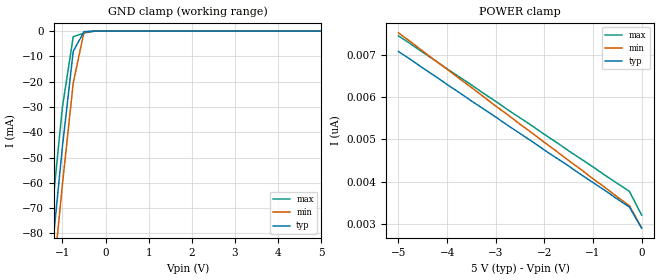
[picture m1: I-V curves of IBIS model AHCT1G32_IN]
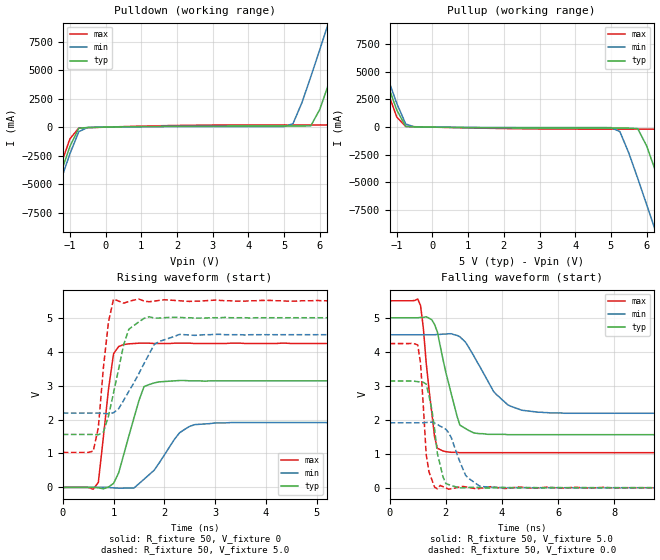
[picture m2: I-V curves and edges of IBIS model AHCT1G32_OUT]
| TEXAS INSTRUMENTS INCORPORATED
| Standard Linear and Logic Group
| IBIS Model of SN74AHCT1G32
| SINGLE 2-INPUT POSITIVE-NOR GATE
| SOT 5-pin (DCK) and SOT 5-pin (DBV) Package
[IBIS Ver]   3.2
[Comment Char]  |_char
[File Name]   ahct1g32.ibs
[File Rev]   2.0 J_die
[Date]   May 24, 2000
[Source]   Data created from HSPICE simulations at TI-SLL.
[Notes]   The following is an IBIS list for the AHCT1G32.
|   Please contact sllibis@ti.com with questions and
|   comments concerning SLL IBIS models.
[Disclaimer] Property of Texas Instruments Incorporated.  Unauthorized
   reproduction and/or distribution is strictly prohibited.
   This product is protected under copyright law.
   Created 2000, (C) Copyright 2000, Texas Instruments Inc.,
   All Rights Reserved.
   UNLESS THERE IS A SIGNED, WRITTEN AGREEMENT TO THE
   CONTRARY, TEXAS INSTRUMENTS () IS PROVIDING THE IBIS
   MODELS  AND WITHOUT ANY WARRANTY, EXPRESSED OR
   IMPLIED.  TI assumes no liability for:
   1) the accuracy of the IBIS models provided to your
   company;
   2) the proper functioning of these IBIS Models in your
   design or for any resulting applications; or
   3) infringement of patents, copyrights or intellectual
   property rights resulting from your use of these IBIS
   models.
   TI provides IBIS Models as a service to our customers.
   You and your company shall not distribute, sell or give
   these models to anyone else without prior written
   permission from TI.
   TI reserves the right to make changes to our products or
   to discontinue any semiconductor product or service
   without notice, and advises our customers to obtain the
   latest version of relevant information to verify, before
   placing orders, that the information being relied on is
   current.
   Please be aware that your receipt and use of the IBIS
   information provided shall serve as acceptance of these
   terms and conditions.  If you do not accept these terms,
   you should return or destroy the IBIS models and any
   other accompanying information immediately.
|   Component AHCT1G32_DCK
[Component]   AHCT1G32_DCK
[Manufacturer]  Texas Instruments, Inc.
[Package]
|   typ   min   max
R_pkg   0.020   0.017   0.025
L_pkg   0.998nH   0.881nH   1.069nH
C_pkg   0.146pF   0.118pF   0.205pF
[Pin]   signal_name   model_name   R_pin   L_pin   C_pin
1   A   AHCT1G32_IN   0.019   1.069nH   0.162pF
2   B   AHCT1G32_IN   0.018   0.881nH   0.121pF
3   GND   GND   0.017   1.031nH   0.205pF
4   Y   AHCT1G32_OUT   0.020   0.960nH   0.124pF
5   VCC   POWER   0.025   1.049nH   0.118pF
|   Component AHCT1G32_DBV
[Component]   AHCT1G32_DBV
[Manufacturer]  Texas Instruments, Inc.
[Package]
|   typ   min   max
R_pkg   0.025   0.021   0.029
L_pkg   1.529nH   1.312nH   1.906nH
C_pkg   0.156pF   0.110pF   0.240pF
[Pin]   signal_name   model_name   R_pin   L_pin   C_pin
1   A   AHCT1G32_IN   0.021   1.511nH   0.144pF
2   B   AHCT1G32_IN   0.023   1.312nH   0.138pF
3   GND   GND   0.029   1.906nH   0.240pF
4   Y   AHCT1G32_OUT   0.026   1.541nH   0.150pF
5   VCC   POWER   0.025   1.374nH   0.110pF
| Models and submodels in the file (2): AHCT1G32_IN (Input), AHCT1G32_OUT (Output)
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|   Model AHCT1G32_IN
[Model]   AHCT1G32_IN
Model_type  Input
Polarity   Inverting
Vinl = 0.8
Vinh = 2.0
| variable   typ   min   max
C_comp   1.24pf   0.93pf   1.55pf
[Temperature Range]   25   85   -40
[Voltage Range]   5.0   4.5   5.5
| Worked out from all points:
|   GND clamp passes 1 mA (typ) near -0.52 V on its own axis
[GND Clamp]
|   Voltage   I(typ)   I(min)   I(max)
-5V       -773mA     -786mA     -758mA
-1.5V     -133mA     -148mA     -117mA
-1.25V    -88.7mA    -104mA     -72.7mA
-1V       -45.6mA    -60.5mA    -30mA
-750mV    -7.99mA    -20.5mA    -2.23mA
-500mV    -233uA     -353uA     -759uA
-250mV    -2.63nA    -182nA     -26.9uA
5V        2.9nA      3.64nA     2.54nA
[POWER Clamp]
|   Voltage   I(typ)   I(min)   I(max)
-5V       7.08nA     7.52nA     7.45nA
-1.5V     4.37nA     4.5nA      4.73nA
-250mV    3.4nA      3.43nA     3.77nA
0V        2.9nA      2.91nA     3.21nA
|   Model AHCT1G32_OUT
[Model]   AHCT1G32_OUT
Model_type  Output
Polarity   Inverting
Vmeas = 2.50v
Cref = 15pf
| variable   typ   min   max
C_comp   3.12pf   2.34pf   3.90pf
[Temperature Range]   25   85   -40
[Voltage Range]   5.0   4.5   5.5
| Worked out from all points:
|   slope of the pulldown table from 0 to 0.75 V, typ, clamps not added: 18.8 ohm
|   slope of the pullup table from 0 to 0.75 V, typ, clamps not added: 25.3 ohm
|   rising waveform, R_fixture 50, V_fixture 0: 20-80 % time 354ps typ, 551ps min, 196ps max; typ from 0 V to 3.14 V
|   falling waveform, R_fixture 50, V_fixture 5.0: 20-80 % time 588ps typ, 1.04ns min, 331ps max; typ from 5 V to 1.56 V
|   rising waveform, R_fixture 50, V_fixture 5.0: 20-80 % time 301ps typ, 507ps min, 170ps max; typ from 1.56 V to 5 V
|   falling waveform, R_fixture 50, V_fixture 0.0: 20-80 % time 361ps typ, 536ps min, 204ps max; typ from 3.14 V to 0 V
[Pulldown]
|   Voltage   I(typ)   I(min)   I(max)
-5V       -40.9A     -41.4A     -40.3A
-1.75V    -8.76A     -9.39A     -8.09A
-1V       -1.69A     -2.33A     -1.02A
-750mV    -95.5mA    -395mA     -80.6mA
5.25V     93.4mA     298mA      192mA
5.75V     116mA      4.42A      192mA
6.25V     3.8A       9.19A      193mA
6.5V      6.17A      11.6A      931mA
6.75V     8.59A      14.1A      3.15A
7.25V     13.5A      19A        7.96A
7.5V      15.9A      21.4A      10.4A
10V       40.7A      46.2A      35.2A
[Pullup]
|   Voltage   I(typ)   I(min)   I(max)
-5V       40.7A      41.2A      40.1A
-2V       11A        11.6A      10.4A
-1.75V    8.59A      9.19A      7.96A
-1V       1.54A      2.14A      907mA
-750mV    63.6mA     284mA      62.5mA
5.25V     -84.4mA    -401mA     -178mA
5.75V     -130mA     -4.62A     -178mA
6.25V     -3.97A     -9.39A     -187mA
6.75V     -8.76A     -14.3A     -3.28A
7.25V     -13.6A     -19.2A     -8.09A
7.5V      -16.1A     -21.6A     -10.5A
10V       -40.9A     -46.4A     -35.3A
[Ramp]
| variable   typ   min   max
dV/dt_r   1.88E+00/3.01E-10   1.16E+00/5.09E-10   2.56E+00/1.64E-10
dV/dt_f   2.09E+00/5.34E-10   1.41E+00/9.86E-10   2.72E+00/2.77E-10
R_load = 50
[Rising Waveform]
R_fixture = 50
V_fixture = 0
|   Time   V(typ)   V(min)   V(max)
0s        0V         0V         0V
600ps     1.55mV     230uV      -52.1mV
700ps     -10.4mV    2.17mV     147mV
900ps     11.1mV     -1.37mV    2.89V
1ns       118mV      -14.2mV    3.94V
1.3ns     1.51V      -20.4mV    4.23V
1.6ns     2.97V      242mV      4.25V
2.3ns     3.15V      1.61V      4.25V
3ns       3.14V      1.9V       4.24V
25ns      3.14V      1.91V      4.24V
[Falling Waveform]
R_fixture = 50
V_fixture = 5.0
V_fixture_min = 4.5
V_fixture_max = 5.5
|   Time   V(typ)   V(min)   V(max)
0s        5V         4.5V       5.5V
1ns       5V         4.5V       5.55V
1.1ns     5.01V      4.5V       5.36V
1.6ns     4.8V       4.5V       1.49V
1.7ns     4.58V      4.51V      1.16V
2ns       3.39V      4.52V      1.06V
2.5ns     1.84V      4.44V      1.03V
3.7ns     1.57V      2.83V      1.03V
4.7ns     1.56V      2.28V      1.03V
25ns      1.56V      2.19V      1.03V
[Rising Waveform]
R_fixture = 50
V_fixture = 5.0
V_fixture_min = 4.5
V_fixture_max = 5.5
|   Time   V(typ)   V(min)   V(max)
0s        1.56V      2.19V      1.03V
600ps     1.56V      2.19V      1.07V
700ps     1.55V      2.19V      1.76V
800ps     1.63V      2.18V      3.53V
900ps     2.1V       2.17V      4.88V
1ns       2.79V      2.2V       5.55V
1.3ns     4.66V      2.83V      5.48V
1.8ns     4.99V      4.21V      5.49V
2.3ns     5.01V      4.51V      5.5V
25ns      5V         4.5V       5.5V
[Falling Waveform]
R_fixture = 50
V_fixture = 0.0
|   Time   V(typ)   V(min)   V(max)
0s        3.14V      1.91V      4.24V
1ns       3.12V      1.91V      4.2V
1.1ns     3.11V      1.91V      3.66V
1.3ns     3.05V      1.92V      976mV
1.5ns     2.31V      1.93V      240mV
1.7ns     1V         1.86V      -31.8mV
2ns       121mV      1.72V      -6.75mV
2.7ns     1.28mV     369mV      25.5mV
3.3ns     -281uV     32mV       -9.27mV
25ns      0V         0V         0V
